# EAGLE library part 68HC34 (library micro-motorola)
MICROCONTROLLER/MEMORY DEVICE
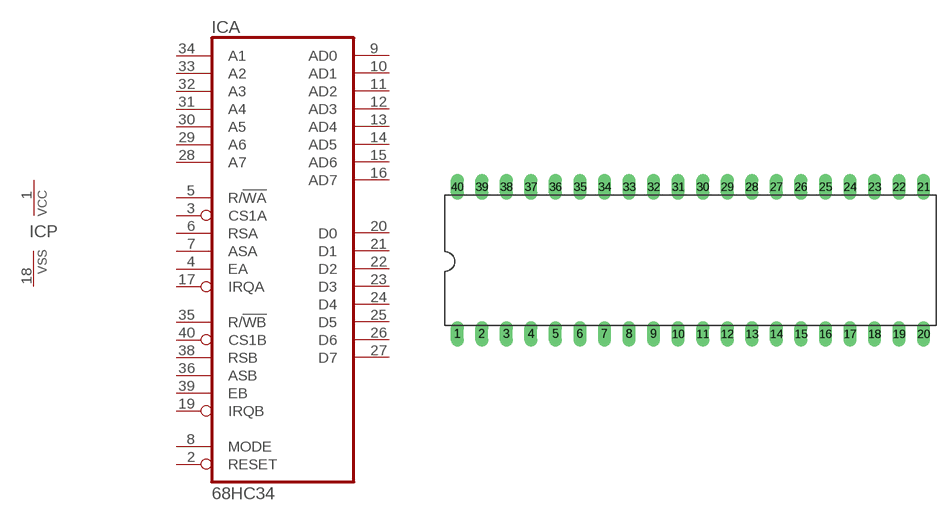
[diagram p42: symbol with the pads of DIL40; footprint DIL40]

Designator prefix IC; gates A=68HC34 P=PWRVSS

## 68HC34 (OC_FARNELL: unknown; OC_NEWARK: unknown)  [DIL40]
1  P:VCC  pwr
2  A:RESET  in
3  A:CS1A  in
4  A:EA  in
5  A:R/!WA  in
6  A:RSA  in
7  A:ASA  in
8  A:MODE  in
9  A:AD0
10  A:AD1
11  A:AD2
12  A:AD3
13  A:AD4
14  A:AD5
15  A:AD6
16  A:AD7
17  A:IRQA  in
18  P:VSS  pwr
19  A:IRQB  in
20  A:D0
21  A:D1
22  A:D2
23  A:D3
24  A:D4
25  A:D5
26  A:D6
27  A:D7
28  A:A7  in
29  A:A6  in
30  A:A5  in
31  A:A4  in
32  A:A3  in
33  A:A2  in
34  A:A1  in
35  A:R/!WB  in
36  A:ASB  in
38  A:RSB  in
39  A:EB  in
40  A:CS1B  in

## Footprint DIL40 (pad centres in mm)
Dual In Line Package
drill 0.813 long: 1 -24.13,-7.62; 2 -21.59,-7.62; 3 -19.05,-7.62; 4 -16.51,-7.62; 5 -13.97,-7.62; 6 -11.43,-7.62; 7 -8.89,-7.62; 8 -6.35,-7.62; 9 -3.81,-7.62; 10 -1.27,-7.62; 11 1.27,-7.62; 12 3.81,-7.62; 13 6.35,-7.62; 14 8.89,-7.62; 15 11.43,-7.62; 16 13.97,-7.62; 17 16.51,-7.62; 18 19.05,-7.62; 19 21.59,-7.62; 20 24.13,-7.62; 21 24.13,7.62; 22 21.59,7.62; 23 19.05,7.62; 24 16.51,7.62; 25 13.97,7.62; 26 11.43,7.62; 27 8.89,7.62; 28 6.35,7.62; 29 3.81,7.62; 30 1.27,7.62; 31 -1.27,7.62; 32 -3.81,7.62; 33 -6.35,7.62; 34 -8.89,7.62; 35 -11.43,7.62; 36 -13.97,7.62; 37 -16.51,7.62; 38 -19.05,7.62; 39 -21.59,7.62; 40 -24.13,7.62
